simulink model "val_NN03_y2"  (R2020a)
settings: Solver=ode45  StartTime=0.0  StopTime=100  RelTol=1e-3  EnableMultiTasking=on
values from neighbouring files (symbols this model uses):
  Ts = 0.05    [init_model.m]
libraries: neural x26

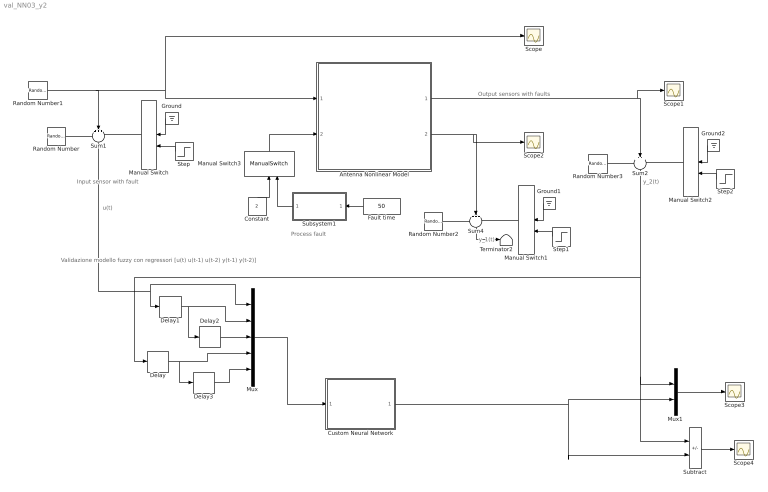
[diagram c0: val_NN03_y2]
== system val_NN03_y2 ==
  note: Validazione modello fuzzy con regressori [u(t) u(t-1) u(t-2) y(t-1) y(t-2)]
  note: u(t)
  note: Output sensors with faults
  note: Process fault
  note: Input sensor with fault
  note: y_1(t)
  note: y_2(t)
  Antenna Nonlinear Model : Subsystem
  Constant : Constant  Value=2
  Custom Neural Network : Subsystem
      mask help: Custom Neural Network
  Delay{,1..3} (4 alike) : Delay  DelayLength=1  SampleTime=Ts
  Fault time : Constant  Value=50
  Ground : Ground
  Ground1 : Ground
  Ground2 : Ground
  Manual Switch : ManualSwitch  CurrentSetting=0
  Manual Switch1 : ManualSwitch
  Manual Switch2 : ManualSwitch
  Manual Switch3 : ManualSwitch
  Mux : Mux  Inputs=5
  Mux1 : Mux  Inputs=2
  Random Number : RandomNumber  Variance=0.0001  Seed=1  SampleTime=Ts
  Random Number1 : RandomNumber  Variance=0.1  SampleTime=10
  Random Number2 : RandomNumber  Variance=0.00001  Seed=2  SampleTime=Ts
  Random Number3 : RandomNumber  Variance=0.00001  Seed=3  SampleTime=Ts
  Scope{,1..4} (5 alike) : Scope
  Step : Step  Time=50  SampleTime=0
  Step1 : Step  Time=50  SampleTime=0
  Step2 : Step  Time=50  SampleTime=0
  Subsystem1 : Subsystem
  Subtract : Sum  Inputs=+-
  Sum1 : Sum  Inputs=+++  SaturateOnIntegerOverflow=on
  Sum2 : Sum  Inputs=+++  SaturateOnIntegerOverflow=on
  Sum4 : Sum  Inputs=+++  SaturateOnIntegerOverflow=on
  Terminator2 : Terminator
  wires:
  Random Number1/1 -> Scope/1, Antenna Nonlinear Model/1(force), Sum1/2
  Random Number/1 -> Sum1/1
  Manual Switch/1 -> Sum1/3
  Sum1/1 -> Delay1/1, Mux/1
  Ground/1 -> Manual Switch/1
  Step/1 -> Manual Switch/2
  Random Number2/1 -> Sum4/1
  Ground1/1 -> Manual Switch1/1
  Manual Switch1/1 -> Sum4/3
  Step1/1 -> Manual Switch1/2
  Antenna Nonlinear Model/2(velocity) -> Sum4/2, Scope2/1
  Random Number3/1 -> Sum2/1
  Ground2/1 -> Manual Switch2/1
  Manual Switch2/1 -> Sum2/3
  Step2/1 -> Manual Switch2/2
  Antenna Nonlinear Model/1(angle) -> Sum2/2, Scope1/1
  Sum2/1 -> Subtract/1, Mux1/1, Delay/1
  Fault time/1 -> Subsystem1/1(Fault time)
  Subsystem1/1(Fault) -> Manual Switch3/2
  Manual Switch3/1 -> Antenna Nonlinear Model/2(drag)
  Constant/1 -> Manual Switch3/1
  Mux/1 -> Custom Neural Network/1(Input)
  Delay1/1 -> Delay2/1, Mux/2
  Delay2/1 -> Mux/3
  Delay/1 -> Delay3/1, Mux/4
  Delay3/1 -> Mux/5
  Custom Neural Network/1(Output) -> Subtract/2, Mux1/2
  Mux1/1 -> Scope3/1
  Subtract/1 -> Scope4/1
  Sum4/1 -> Terminator2/1

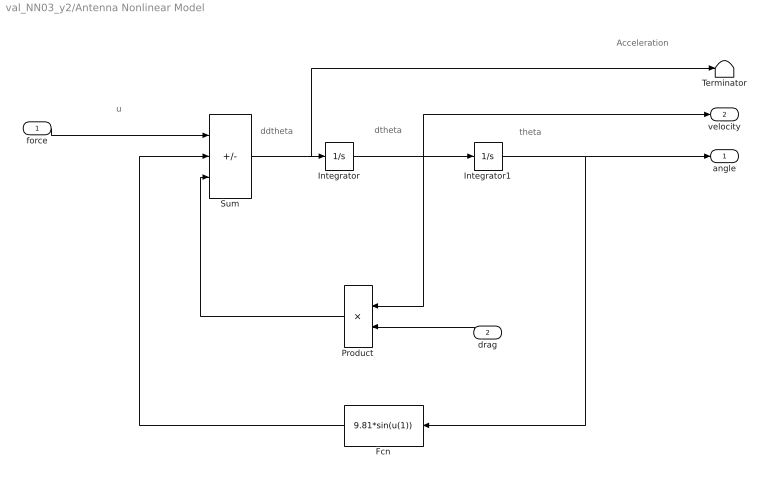
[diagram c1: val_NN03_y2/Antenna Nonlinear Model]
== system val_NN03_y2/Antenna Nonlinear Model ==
  note: Acceleration
  note: ddtheta
  note: dtheta
  note: theta
  note: u
  force : Inport
  drag : Inport  Port=2
  Fcn : Fcn  Expr=9.81*sin(u(1))
  Integrator : Integrator
  Integrator1 : Integrator  InitialCondition=(pi/180)*90
  Product : Product
  Sum : Sum  Inputs=+--  SaturateOnIntegerOverflow=on
  Terminator : Terminator
  angle : Outport
  velocity : Outport  Port=2
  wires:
  Sum/1 -> Terminator/1, Integrator/1
  Integrator/1 -> Product/1, Integrator1/1, velocity/1
  Integrator1/1 -> angle/1, Fcn/1
  Fcn/1 -> Sum/2
  Product/1 -> Sum/3
  force/1 -> Sum/1
  drag/1 -> Product/2

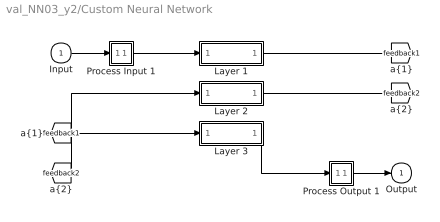
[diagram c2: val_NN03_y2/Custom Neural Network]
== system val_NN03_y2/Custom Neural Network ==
  Input : Inport  PortDimensions=5  SampleTime=0.05
  Layer 1 : Subsystem
  Layer 2 : Subsystem
  Layer 3 : Subsystem
  Process Input 1 : Subsystem
  Process Output 1 : Subsystem
  Output : Outport  InitialOutput=0
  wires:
  Input/1 -> Process Input 1/1(x)
  Process Output 1/1(y) -> Output/1
  Process Input 1/1(p) -> Layer 1/1("p{1}")
  Layer 1/1("a{1}") -> [feedback1]
  [feedback1] -> Layer 2/1("a{1} ")
  Layer 2/1("a{2}") -> [feedback2]
  [feedback2] -> Layer 3/1("a{2} ")
  Layer 3/1("a{3}") -> Process Output 1/1(a)

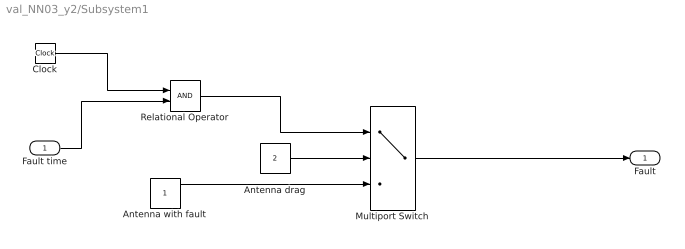
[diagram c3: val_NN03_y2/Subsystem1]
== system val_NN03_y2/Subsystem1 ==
  Fault time : Inport
  Antenna drag : Constant  Value=2
  Antenna with fault : Constant
  Clock : Clock
  Multiport Switch : MultiPortSwitch  DataPortOrder=Zero-based contiguous  Inputs=2  zeroidx=on
  Relational Operator : RelationalOperator  OutDataTypeStr=boolean  RndMeth=Simplest
  Fault : Outport
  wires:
  Clock/1 -> Relational Operator/1
  Fault time/1 -> Relational Operator/2
  Antenna drag/1 -> Multiport Switch/2
  Relational Operator/1 -> Multiport Switch/1
  Multiport Switch/1 -> Fault/1
  Antenna with fault/1 -> Multiport Switch/3

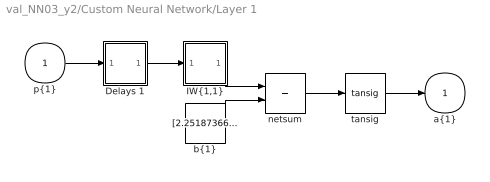
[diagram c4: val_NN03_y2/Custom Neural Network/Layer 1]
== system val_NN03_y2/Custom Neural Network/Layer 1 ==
  "p{1}" : Inport  PortDimensions=5  SampleTime=0.05
  Delays 1 : Subsystem
  "IW{1,1}" : Subsystem
  "b{1}" : Constant  Value=[2.251873667793956368399221901199780404567718505859375;0.9242637528006591995932694771909154951572418212890625;-0.031071950679221214952629992467336705885827541351318359375;1.114833352237121655292639843537472188472747802734375;-0.84478619087160378153811279844376258552074432373046875;-1.4914147804270305730511836372897960245609283447265625;-3.8327323367625805161651442176662385463714599609375]
  netsum : Sum  Inputs=2  InputSameDT=on  SaturateOnIntegerOverflow=on
  tansig : neural/Transfer Functions/tansig
  "a{1}" : Outport  InitialOutput=[0;0;0;0;0;0;0]
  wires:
  "p{1}"/1 -> Delays 1/1("p{1}")
  Delays 1/1("pd{1,1}") -> "IW{1,1}"/1("pd{1,1}")
  "IW{1,1}"/1("iz{1,1}") -> netsum/1
  "b{1}"/1 -> netsum/2
  netsum/1 -> tansig/1
  tansig/1 -> "a{1}"/1

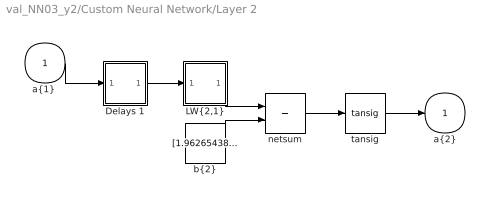
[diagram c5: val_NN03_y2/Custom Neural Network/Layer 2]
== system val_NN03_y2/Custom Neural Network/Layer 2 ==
  "a{1} " : Inport  PortDimensions=7  SampleTime=0.05
  Delays 1 : Subsystem
  "LW{2,1}" : Subsystem
  "b{2}" : Constant  Value=[1.9626543834130989463204741696245037019252777099609375;1.859400253425581350796846891171298921108245849609375;-1.661922883162452624361549169407226145267486572265625;-1.4298736668650986469941699397168122231960296630859375;0.84353592584759040651221084772259928286075592041015625;-0.57314502311066906070635695868986658751964569091796875;-0.264434440066442288941317428907495923340320587158203125;0.118265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
  netsum : Sum  Inputs=2  InputSameDT=on  SaturateOnIntegerOverflow=on
  tansig : neural/Transfer Functions/tansig
  "a{2}" : Outport  InitialOutput=[0;0;0;0;0;0;0;0;0;0;0;0;0;0;0]
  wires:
  "a{1} "/1 -> Delays 1/1("p{2}")
  Delays 1/1("pd{2,1}") -> "LW{2,1}"/1("ad{2,1}")
  "LW{2,1}"/1("lz{2,1}") -> netsum/1
  "b{2}"/1 -> netsum/2
  netsum/1 -> tansig/1
  tansig/1 -> "a{2}"/1

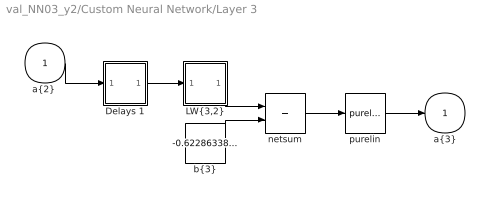
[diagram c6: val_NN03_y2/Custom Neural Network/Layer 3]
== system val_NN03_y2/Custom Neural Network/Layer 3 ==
  "a{2} " : Inport  PortDimensions=15  SampleTime=0.05
  Delays 1 : Subsystem
  "LW{3,2}" : Subsystem
  "b{3}" : Constant  Value=-0.62286338353077363994003690095269121229648590087890625
  netsum : Sum  Inputs=2  InputSameDT=on  SaturateOnIntegerOverflow=on
  purelin : neural/Transfer Functions/purelin
  "a{3}" : Outport  InitialOutput=0
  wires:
  "a{2} "/1 -> Delays 1/1("p{3}")
  Delays 1/1("pd{3,2}") -> "LW{3,2}"/1("ad{3,2}")
  "LW{3,2}"/1("lz{3,2}") -> netsum/1
  "b{3}"/1 -> netsum/2
  netsum/1 -> purelin/1
  purelin/1 -> "a{3}"/1

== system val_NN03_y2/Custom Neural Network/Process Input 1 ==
  x : Inport  PortDimensions=5  SampleTime=0.05
  p : Outport  PortDimensions=5  SampleTime=0.05
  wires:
  x/1 -> p/1

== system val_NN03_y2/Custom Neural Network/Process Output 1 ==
  a : Inport  PortDimensions=1  SampleTime=0.05
  y : Outport  PortDimensions=1  SampleTime=0.05
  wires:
  a/1 -> y/1

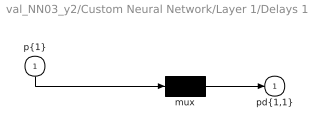
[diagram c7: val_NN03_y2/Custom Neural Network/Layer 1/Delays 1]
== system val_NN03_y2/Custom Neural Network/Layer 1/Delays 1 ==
  "p{1}" : Inport  PortDimensions=5  SampleTime=0.05
  mux : Mux  Inputs=1
  "pd{1,1}" : Outport
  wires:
  "p{1}"/1 -> mux/1
  mux/1 -> "pd{1,1}"/1

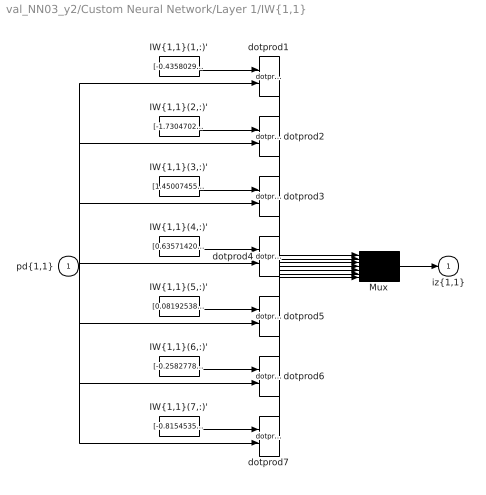
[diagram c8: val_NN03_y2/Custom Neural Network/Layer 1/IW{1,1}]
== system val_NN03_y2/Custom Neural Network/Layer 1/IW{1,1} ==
  "pd{1,1}" : Inport  PortDimensions=5  SampleTime=0.05
  "IW{1,1}(1,:)'" : Constant  Value=[-0.435802941743758942561015601313556544482707977294921875;1.7872812573833625204855479751131497323513031005859375;-1.764592682163569126174706980236805975437164306640625;-0.404377003020619019135750704663223586976528167724609375;0.52534178623082661285792482885881327092647552490234375]
  "IW{1,1}(2,:)'" : Constant  Value=[-1.730470219024559330733836759463883936405181884765625;0.151640285788593953686387294510495848953723907470703125;-1.2905899460165761727381550372228957712650299072265625;1.2644484505864543866238136615720577538013458251953125;0.1848876989484178057221441804358619265258312225341796875]
  "IW{1,1}(3,:)'" : Constant  Value=[1.45007455733940648912039250717498362064361572265625;-0.7561060804104904331524039662326686084270477294921875;1.1553895245046066353467040244140662252902984619140625;0.045456691390366878169349007521304883994162082672119140625;0.78795900054040679538758240596507675945758819580078125]
  "IW{1,1}(4,:)'" : Constant  Value=[0.6357142071010404293929241248406469821929931640625;0.615633947993070140825011549168266355991363525390625;1.35771096878878250180378017830662429332733154296875;-1.325505954824133691971610460313968360424041748046875;-0.03528837958723786416559420331395813263952732086181640625]
  "IW{1,1}(5,:)'" : Constant  Value=[0.0819253886907822248542032639306853525340557098388671875;-0.5064268106985798656438646503374911844730377197265625;0.37060122805194328776678958092816174030303955078125;-1.736018131141083831181504137930460274219512939453125;0.81382200422844130915933646974735893309116363525390625]
  "IW{1,1}(6,:)'" : Constant  Value=[-0.258277855514971566019966076055425219237804412841796875;-1.01821335927758749306804020307026803493499755859375;-1.7617609560684004410546776853152550756931304931640625;0.74180349939032053097065499969176016747951507568359375;-1.1683533816478506306424378635711036622524261474609375]
  "IW{1,1}(7,:)'" : Constant  Value=[-0.8154535120297641270781241473741829395294189453125;-0.348912811521184640373149932202068157494068145751953125;-1.4230719993131664136143399446154944598674774169921875;0.884253756502624721491656600846908986568450927734375;0.7082996790592754887683213382842950522899627685546875]
  Mux : Mux  Inputs=7
  dotprod{1..7} (7 alike) : neural/Weight Functions/dotprod
  "iz{1,1}" : Outport
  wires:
  "IW{1,1}(1,:)'"/1 -> dotprod1/1
  "pd{1,1}"/1 -> dotprod1/2, dotprod2/2, dotprod3/2, dotprod4/2, dotprod5/2, dotprod6/2, dotprod7/2
  dotprod1/1 -> Mux/1
  "IW{1,1}(2,:)'"/1 -> dotprod2/1
  dotprod2/1 -> Mux/2
  "IW{1,1}(3,:)'"/1 -> dotprod3/1
  dotprod3/1 -> Mux/3
  "IW{1,1}(4,:)'"/1 -> dotprod4/1
  dotprod4/1 -> Mux/4
  "IW{1,1}(5,:)'"/1 -> dotprod5/1
  dotprod5/1 -> Mux/5
  "IW{1,1}(6,:)'"/1 -> dotprod6/1
  dotprod6/1 -> Mux/6
  "IW{1,1}(7,:)'"/1 -> dotprod7/1
  dotprod7/1 -> Mux/7
  Mux/1 -> "iz{1,1}"/1

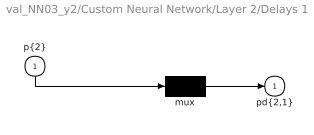
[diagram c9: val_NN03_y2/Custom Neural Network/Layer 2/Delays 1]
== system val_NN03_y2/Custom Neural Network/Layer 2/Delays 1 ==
  "p{2}" : Inport  PortDimensions=7  SampleTime=0.05
  mux : Mux  Inputs=1
  "pd{2,1}" : Outport
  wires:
  "p{2}"/1 -> mux/1
  mux/1 -> "pd{2,1}"/1

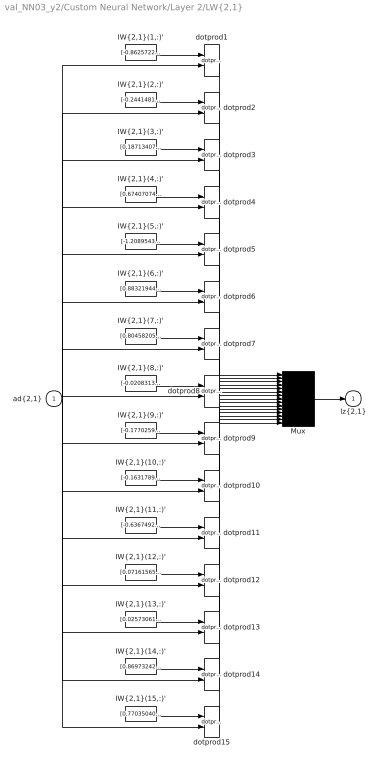
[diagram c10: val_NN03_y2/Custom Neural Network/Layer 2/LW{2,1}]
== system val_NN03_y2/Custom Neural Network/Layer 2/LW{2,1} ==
  "ad{2,1}" : Inport  PortDimensions=7  SampleTime=0.05
  "IW{2,1}(1,:)'" : Constant  Value=[-0.8625722358742546891363645045203156769275665283203125;0.2743133773136656738955707623972557485103607177734375;-0.7226016493302294119160933405510149896144866943359375;0.323387432416578246563432230686885304749011993408203125;0.67327789326867681918287189546390436589717864990234375;-1.3107234322884602217840210869326256215572357177734375;1.03127373412379430561713888891972601413726806640625]
  "IW{2,1}(10,:)'" : Constant  Value=[-0.1631789298797725329404073590922052972018718719482421875;0.31395381603033800654856122491764836013317108154296875;1.3356308085669061913591804113821126520633697509765625;0.052052402475086793909309079708691569976508617401123046875;-0.040237511831074400381336175769320107065141201019287109375;0.743515154493579633054878286202438175678253173828125;1.3229667984852457873756748085725121200084686279296875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
  "IW{2,1}(11,:)'" : Constant  Value=[-0.63674920143391045002090322668664157390594482421875;-0.6528669963421342981035877528483979403972625732421875;0.89775734910930571341936001772410236299037933349609375;-0.91819219079162817109818206517957150936126708984375;0.57242445657157914329360437477589584887027740478515625;-0.776153650737032574369322901475243270397186279296875;0.454106084634724960213958411259227432310581207275390625]
  "IW{2,1}(12,:)'" : Constant  Value=[0.0716156519478554631774613881134428083896636962890625;-1.034856112150081219880348726292140781879425048828125;-0.301267038742567938580663167158490978181362152099609375;-1.1933924812712743968035056241205893456935882568359375;0.830179452138637419267297445912845432758331298828125;0.77224958101109197894373892268049530684947967529296875;0.5695123864539477498425412704818882048130035400390625]
  "IW{2,1}(13,:)'" : Constant  Value=[0.025730611241079094642092428557589300908148288726806640625;-0.054619228076915160574600349718821235001087188720703125;-1.4096475723363737220239499947638250887393951416015625;1.25613367086818872309095240780152380466461181640625;-0.177730645219068505991089068629662506282329559326171875;0.07662542591365238686673677648286684416234493255615234375;1.133094868830405221871160392765887081623077392578125]
  "IW{2,1}(14,:)'" : Constant  Value=[0.86973242016059615355771938993711955845355987548828125;-0.53793864953700831765814882601262070238590240478515625;-0.3366562259393253153660907628363929688930511474609375;-1.1311819301949654903438613473554141819477081298828125;-0.197995002609133885496106586288078688085079193115234375;0.790994073620737925267576429178006947040557861328125;0.68860884579803294247568601349485106766223907470703125]
  "IW{2,1}(15,:)'" : Constant  Value=[0.77035040088569528560213939272216521203517913818359375;0.88163843309972766970616930848336778581142425537109375;-0.2181613604302469477946857523420476354658603668212890625;1.0543472211380493508414701864239759743213653564453125;1.1719319647314871968291072334977798163890838623046875;0.49706193152707955906777215204783715307712554931640625;0.1511387032512624684077451320263207890093326568603515625]
  "IW{2,1}(2,:)'" : Constant  Value=[-0.2441481327956891711483677909200196154415607452392578125;-0.26685166179733699198806107233394868671894073486328125;-0.8859363073484132211632413600455038249492645263671875;-0.75748120079157710282657944844686426222324371337890625;-0.0076520819378477454575371297096353373490273952484130859375;1.26338766283201575646444325684569776058197021484375;1.08613797022568814298892903025262057781219482421875]
  "IW{2,1}(3,:)'" : Constant  Value=[0.1871340717506138895398493104949011467397212982177734375;0.69792042029859502338950960620422847568988800048828125;-1.0809646357565612095896767641534097492694854736328125;0.328954593116599303126434961086488328874111175537109375;0.00662213199911958379229037774393873405642807483673095703125;0.93455381414267602036005655463668517768383026123046875;-0.298641652770060772592586317841778509318828582763671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
  "IW{2,1}(4,:)'" : Constant  Value=[0.674070743928206095318955703987739980220794677734375;0.061009478407589849691117223073888453654944896697998046875;-0.54180390811614109747296197383548133075237274169921875;0.476473023658479821751399185814079828560352325439453125;-0.45167415543771072261591825736104510724544525146484375;1.1396355791005021718120815421571023762226104736328125;0.775423544819404231276394057204015552997589111328125]
  "IW{2,1}(5,:)'" : Constant  Value=[-1.208954357037416826869957731105387210845947265625;-0.4752058598368218422791642296942882239818572998046875;-0.2367764633828361720002675383511814288794994354248046875;-0.7832840827291518426278571496368385851383209228515625;-0.081929945558525674176308939422597177326679229736328125;-1.0883366102590306123687469153082929551601409912109375;-0.790736589964381675343929600785486400127410888671875]
  "IW{2,1}(6,:)'" : Constant  Value=[0.883219440464975580340478700236417353153228759765625;0.65832450145922172257684223950491286814212799072265625;0.22020490939265957575088350495207123458385467529296875;-0.60577646498878079395211670998833142220973968505859375;1.0502341688241330075470614247024059295654296875;-0.57548136187187626244821103682625107467174530029296875;-1.000389618685450177082429945585317909717559814453125]
  "IW{2,1}(7,:)'" : Constant  Value=[0.804582059858976794686213906970806419849395751953125;0.76359736744918638162715751604991964995861053466796875;0.7634400422189544510587211334495805203914642333984375;-0.405577801412497385147304385100142098963260650634765625;-0.169586443608446824082847115278127603232860565185546875;-0.64130077060436097013962353230454027652740478515625;0.8022784945839604997530614127754233777523040771484375]
  "IW{2,1}(8,:)'" : Constant  Value=[-0.0208313239033162365954066075346418074332177639007568359375;0.51512857296853031829897417992469854652881622314453125;-0.428043104743494884356636021038866601884365081787109375;-1.35374545462782780447241748333908617496490478515625;0.01482348429886731246141184925591005594469606876373291015625;1.0996817145657364900301899979240261018276214599609375;-0.1145707497407440350611906865196942817419767379760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
  "IW{2,1}(9,:)'" : Constant  Value=[-0.1770259108469489361947779570982675068080425262451171875;0.26007362466071326512206951520056463778018951416015625;-1.1052272285418516251098708380595780909061431884765625;-0.4199344695841915608980343677103519439697265625;-0.89820749927333942697060820137267000973224639892578125;-1.05842682331720983057721241493709385395050048828125;-0.06809334755198659383523818178218789398670196533203125]
  Mux : Mux  Inputs=15
  dotprod{1..15} (15 alike) : neural/Weight Functions/dotprod
  "lz{2,1}" : Outport
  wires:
  "IW{2,1}(1,:)'"/1 -> dotprod1/1
  "ad{2,1}"/1 -> dotprod1/2, dotprod2/2, dotprod3/2, dotprod4/2, dotprod5/2, dotprod6/2, dotprod7/2, dotprod8/2, dotprod9/2, dotprod10/2, dotprod11/2, dotprod12/2, dotprod13/2, dotprod14/2, dotprod15/2
  dotprod1/1 -> Mux/1
  "IW{2,1}(2,:)'"/1 -> dotprod2/1
  dotprod2/1 -> Mux/2
  "IW{2,1}(3,:)'"/1 -> dotprod3/1
  dotprod3/1 -> Mux/3
  "IW{2,1}(4,:)'"/1 -> dotprod4/1
  dotprod4/1 -> Mux/4
  "IW{2,1}(5,:)'"/1 -> dotprod5/1
  dotprod5/1 -> Mux/5
  "IW{2,1}(6,:)'"/1 -> dotprod6/1
  dotprod6/1 -> Mux/6
  "IW{2,1}(7,:)'"/1 -> dotprod7/1
  dotprod7/1 -> Mux/7
  "IW{2,1}(8,:)'"/1 -> dotprod8/1
  dotprod8/1 -> Mux/8
  "IW{2,1}(9,:)'"/1 -> dotprod9/1
  dotprod9/1 -> Mux/9
  "IW{2,1}(10,:)'"/1 -> dotprod10/1
  dotprod10/1 -> Mux/10
  "IW{2,1}(11,:)'"/1 -> dotprod11/1
  dotprod11/1 -> Mux/11
  "IW{2,1}(12,:)'"/1 -> dotprod12/1
  dotprod12/1 -> Mux/12
  "IW{2,1}(13,:)'"/1 -> dotprod13/1
  dotprod13/1 -> Mux/13
  "IW{2,1}(14,:)'"/1 -> dotprod14/1
  dotprod14/1 -> Mux/14
  "IW{2,1}(15,:)'"/1 -> dotprod15/1
  dotprod15/1 -> Mux/15
  Mux/1 -> "lz{2,1}"/1

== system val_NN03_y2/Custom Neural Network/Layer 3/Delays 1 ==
  "p{3}" : Inport  PortDimensions=15  SampleTime=0.05
  mux : Mux  Inputs=1
  "pd{3,2}" : Outport
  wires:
  "p{3}"/1 -> mux/1
  mux/1 -> "pd{3,2}"/1

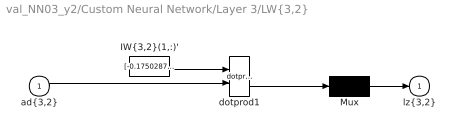
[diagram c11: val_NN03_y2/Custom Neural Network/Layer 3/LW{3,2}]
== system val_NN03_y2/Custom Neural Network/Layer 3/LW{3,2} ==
  "ad{3,2}" : Inport  PortDimensions=15  SampleTime=0.05
  "IW{3,2}(1,:)'" : Constant  Value=[-0.175028750502748631223681741175823844969272613525390625;-0.5297119573505550960135224158875644207000732421875;0.428624086766544343252149928957805968821048736572265625;-0.287940858640388819278399523682310245931148529052734375;0.1308082733611585501964924560525105334818363189697265625;-0.48670606710422992247089268857962451875209808349609375;0.350111871623175530121585552478791214525699615478515625;0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
  Mux : Mux  Inputs=1
  dotprod1 : neural/Weight Functions/dotprod
  "lz{3,2}" : Outport
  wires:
  "IW{3,2}(1,:)'"/1 -> dotprod1/1
  "ad{3,2}"/1 -> dotprod1/2
  dotprod1/1 -> Mux/1
  Mux/1 -> "lz{3,2}"/1
